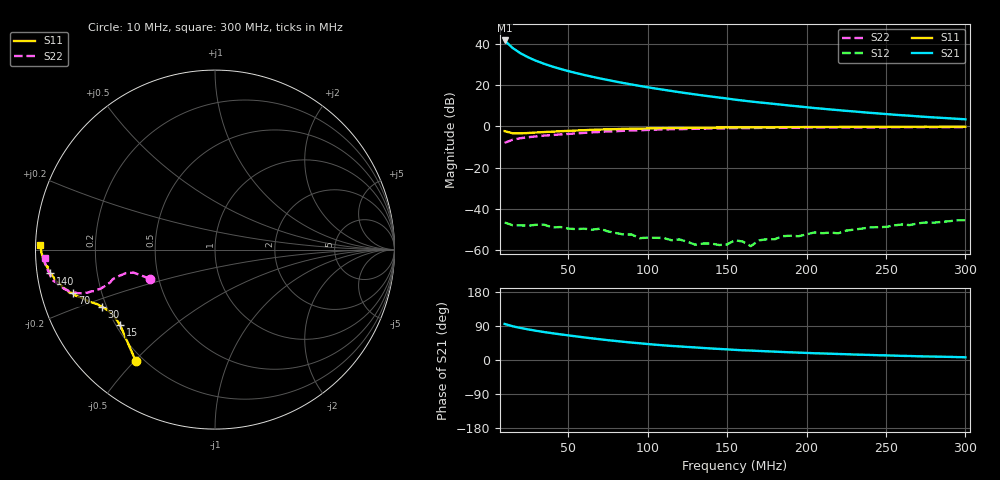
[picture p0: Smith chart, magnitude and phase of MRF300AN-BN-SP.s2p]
! Copyright - 2018 NXP B.V.
! 05/31/2018
! Rev 0
! MRF300AN/BN S-Parameters
! Vdd=50 V, IDQ=1000 mA
# hz S ma R 50
! Comment
! freq  magS11  angS11  magS21  angS21  magS12  angS12  magS22  angS22
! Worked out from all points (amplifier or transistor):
!   59 points, 10 MHz to 300 MHz, reference 50 ohm
!   highest |S21| = 41.6 dB at 10 MHz (marker M1)
!   |S21| within 3 dB of that: start of sweep to 14.15 MHz
!   unconditionally stable (mu >= 1): 38.8 MHz to 68.37 MHz; 72.18 MHz to 153.9 MHz; 157 MHz to 181.5 MHz
!   at 55 MHz: K = 1.18, MAG = 35.3 dB, |S12| = -49.8 dB
!   at 155 MHz: K = 0.90, MSG = 34.0 dB, |S12| = -55.2 dB
!   at 300 MHz: K = 0.32, MSG = 24.5 dB, |S12| = -45.5 dB
!   S11 on the Smith chart (normalised r, x): 10 MHz: 0.17, -0.50; 15 MHz: 0.22, -0.34; 30 MHz: 0.18, -0.23; 70 MHz: 0.10, -0.15; 140 MHz: 0.04, -0.07; 300 MHz: 0.01, +0.01
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1e7  0.7612 -125.5  119.8 95.2  0.004664 0.7  0.3964 -155.7
1.5e7  0.6758 -141.5  79.02 89.1  0.004003 1.9  0.4709 -164.2
2e7  0.6732 -147.3  58.55 84.5  0.003974 0.0  0.5137 -165.2
2.5e7  0.6868 -150.5  46.43 80.7  0.003908 0.3  0.5437 -164.8
3e7  0.7069 -153.3  38.27 77.0  0.00411 -3.5  0.5701 -164.4
3.5e7  0.7247 -155.3  32.45 73.7  0.004129 -7.6  0.5939 -163.8
4e7  0.7385 -156.2  28.03 70.7  0.003517 -10.0  0.6112 -162.7
4.5e7  0.7584 -157.6  24.56 67.7  0.003627 -9.4  0.6348 -162.0
5e7  0.7715 -158.7  21.75 65.0  0.003321 -15.2  0.6516 -161.6
5.5e7  0.7865 -159.8  19.46 62.4  0.003224 -17.8  0.6708 -161.2
6e7  0.8035 -160.9  17.51 59.7  0.003305 -18.7  0.691 -161.1
7e7  0.8295 -163.0  14.41 54.8  0.003295 -19.7  0.7283 -161.4
8e7  0.8516 -164.5  12.08 50.2  0.00259 -21.2  0.7594 -161.5
9e7  0.8717 -166.1  10.26 45.9  0.002385 -13.9  0.7906 -162.1
1.1e8  0.9024 -168.7  7.662 38.7  0.001972 10.5  0.84 -163.6
1.25e8  0.9135 -170.4  6.277 34.4  0.001586 -1.5  0.8595 -164.9
1.4e8  0.9271 -171.8  5.245 30.4  0.001446 35.4  0.8826 -166.2
1.55e8  0.9362 -173.4  4.416 26.7  0.001738 32.4  0.8991 -167.8
1.65e8  0.9356 -174.1  3.974 24.9  0.001245 49.9  0.9038 -168.4
2.05e8  0.9586 -176.9  2.762 17.9  0.002672 70.7  0.9302 -171.4
2.55e8  0.9685 -179.6  1.907 11.6  0.003964 80.5  0.945 -174.6
3e8  0.9735 178.4  1.476 7.2  0.00528 83.6  0.951 -177.1
